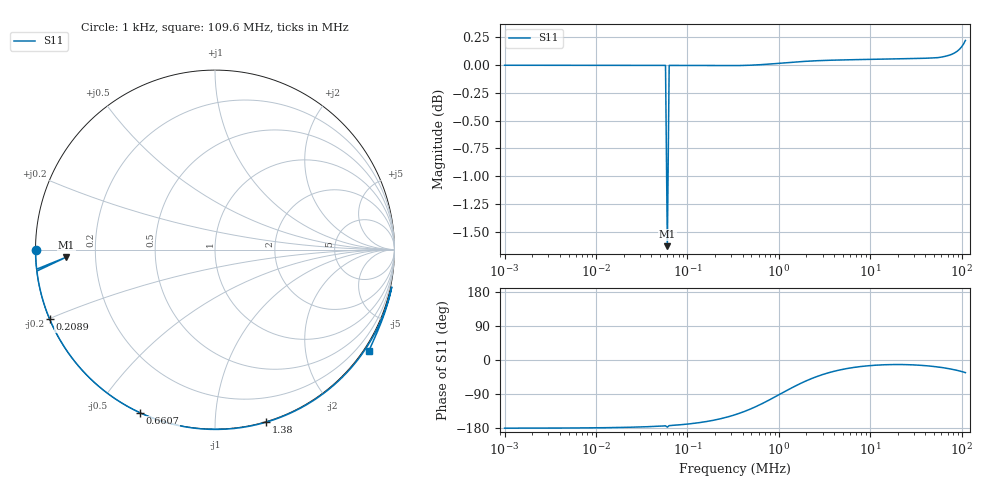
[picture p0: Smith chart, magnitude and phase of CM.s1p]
! EM Consulting and Software
! Touchstone file was created on 2026-03-05  19:00:34
# HZ S RI R 50.0000
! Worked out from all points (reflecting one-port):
!   253 points, 1 kHz to 109.6 MHz, reference 50 ohm
!   lowest |S11| = -1.6 dB at 60.26 kHz (marker M1), VSWR 10.70, Z = 4.68 - j1.25 ohm
!   phase of S11 starts at -180 deg and turns +147 deg over the sweep
!   S11 on the Smith chart (normalised r, x): 1 kHz: 0.00, -0.00; 208.9 kHz: 0.00, -0.20; 660.7 kHz: -0.00, -0.64; 1.38 MHz: -0.00, -1.34; 109.6 MHz: -0.16, -3.34
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1000  -0.9998 -0.00186
4365.158  -0.9998 -0.0082
18197.01  -0.9992 -0.0343
57543.99  -0.9937 -0.1089
60255.96  -0.828 -0.0419
63095.73  -0.9925 -0.1195
79432.82  -0.9882 -0.1505
131825.7  -0.9681 -0.2487
208929.6  -0.9216 -0.3865
331131.1  -0.8138 -0.5802
478630.1  -0.6462 -0.7629
660693.4  -0.4182 -0.9089
954992.6  -0.0761 -0.9988
1148154  0.1076 -0.9965
1380384  0.2841 -0.9618
1445440  0.3258 -0.9487
1995262  0.5777 -0.8211
2754229  0.7519 -0.6663
3981072  0.8705 -0.5024
6025596  0.9382 -0.3618
8317638  0.9641 -0.2867
1.202264e7  0.9787 -0.2334
1.737801e7  0.9843 -0.21
2.630268e7  0.9831 -0.2166
3.981072e7  0.9733 -0.2587
5.754399e7  0.9526 -0.3296
8.317638e7  0.9119 -0.4401
1.096478e8  0.8577 -0.5627
